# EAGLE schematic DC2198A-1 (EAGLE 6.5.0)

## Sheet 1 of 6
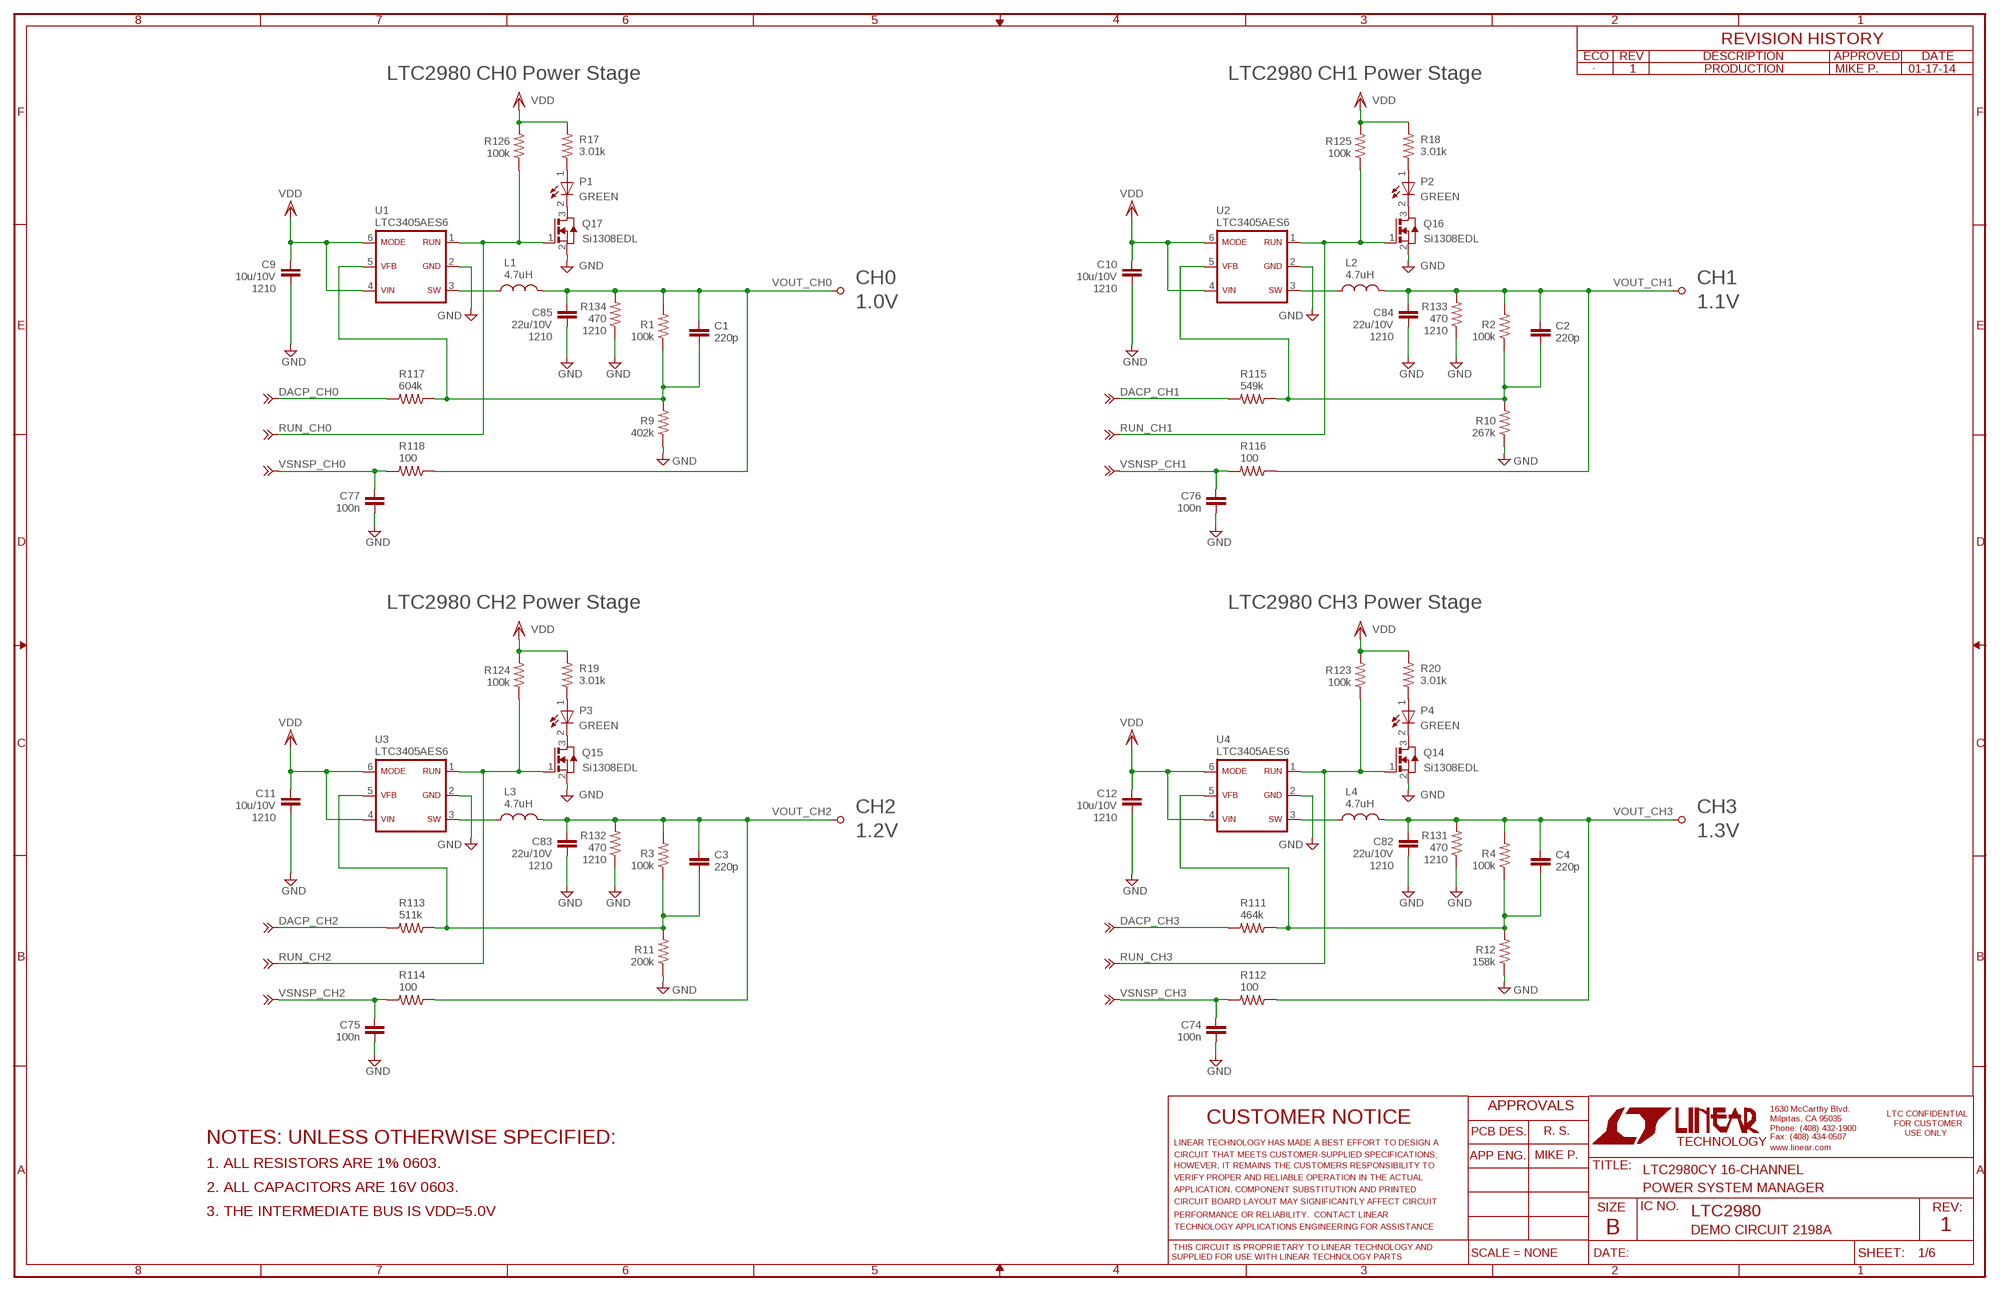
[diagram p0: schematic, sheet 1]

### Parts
C1  220p  CC0603_BOX  [C0603_BOX]
C2  220p  CC0603_BOX  [C0603_BOX]
C3  220p  CC0603_BOX  [C0603_BOX]
C4  220p  CC0603_BOX  [C0603_BOX]
C9  10u/10V  CC1210_BOX  [C1210_BOX]
C10  10u/10V  CC1210_BOX  [C1210_BOX]
C11  10u/10V  CC1210_BOX  [C1210_BOX]
C12  10u/10V  CC1210_BOX  [C1210_BOX]
C74  100n  CC0603_BOX  [C0603_BOX]
C75  100n  CC0603_BOX  [C0603_BOX]
C76  100n  CC0603_BOX  [C0603_BOX]
C77  100n  CC0603_BOX  [C0603_BOX]
C82  22u/10V  CC1210_BOX  [C1210_BOX]
C83  22u/10V  CC1210_BOX  [C1210_BOX]
C84  22u/10V  CC1210_BOX  [C1210_BOX]
C85  22u/10V  CC1210_BOX  [C1210_BOX]
L1  4.7uH  LL1210  [L1210]
L2  4.7uH  LL1210  [L1210]
L3  4.7uH  LL1210  [L1210]
L4  4.7uH  LL1210  [L1210]
P1  GREEN  LED-0603  [CHIPLED_0603]
P2  GREEN  LED-0603  [CHIPLED_0603]
P3  GREEN  LED-0603  [CHIPLED_0603]
P4  GREEN  LED-0603  [CHIPLED_0603]
Q14  Si1308EDL  SI1304  [SC70-3]
Q15  Si1308EDL  SI1304  [SC70-3]
Q16  Si1308EDL  SI1304  [SC70-3]
Q17  Si1308EDL  SI1304  [SC70-3]
R1  100k  RR0603_BOX  [R0603_BOX]
R2  100k  RR0603_BOX  [R0603_BOX]
R3  100k  RR0603_BOX  [R0603_BOX]
R4  100k  RR0603_BOX  [R0603_BOX]
R9  402k  RR0603_BOX  [R0603_BOX]
R10  267k  RR0603_BOX  [R0603_BOX]
R11  200k  RR0603_BOX  [R0603_BOX]
R12  158k  RR0603_BOX  [R0603_BOX]
R17  3.01k  RR0603_BOX  [R0603_BOX]
R18  3.01k  RR0603_BOX  [R0603_BOX]
R19  3.01k  RR0603_BOX  [R0603_BOX]
R20  3.01k  RR0603_BOX  [R0603_BOX]
R111  464k  RR0603_BOX  [R0603_BOX]
R112  100  RR0603_BOX  [R0603_BOX]
R113  511k  RR0603_BOX  [R0603_BOX]
R114  100  RR0603_BOX  [R0603_BOX]
R115  549k  RR0603_BOX  [R0603_BOX]
R116  100  RR0603_BOX  [R0603_BOX]
R117  604k  RR0603_BOX  [R0603_BOX]
R118  100  RR0603_BOX  [R0603_BOX]
R123  100k  RR0603_BOX  [R0603_BOX]
R124  100k  RR0603_BOX  [R0603_BOX]
R125  100k  RR0603_BOX  [R0603_BOX]
R126  100k  RR0603_BOX  [R0603_BOX]
R131  470  RR1210_BOX  [R1210_BOX]
R132  470  RR1210_BOX  [R1210_BOX]
R133  470  RR1210_BOX  [R1210_BOX]
R134  470  RR1210_BOX  [R1210_BOX]
TP3  TESTPOINT_BIG  [TP1]
TP4  TESTPOINT_BIG  [TP1]
TP5  TESTPOINT_BIG  [TP1]
TP6  TESTPOINT_BIG  [TP1]
U1  LTC3405AES6  LTC3405ES6  [SOT-23-6]
U2  LTC3405AES6  LTC3405ES6  [SOT-23-6]
U3  LTC3405AES6  LTC3405ES6  [SOT-23-6]
U4  LTC3405AES6  LTC3405ES6  [SOT-23-6]
VSNSN1  TESPOINT_SMD  TESPOINT_SMDVIA  [VIA]
VSNSN2  TESPOINT_SMD  TESPOINT_SMDVIA  [VIA]
VSNSN3  TESPOINT_SMD  TESPOINT_SMDVIA  [VIA]
VSNSN4  TESPOINT_SMD  TESPOINT_SMDVIA  [VIA]
VSNSN41  TESPOINT_SMD  TESPOINT_SMDVIA  [VIA]
VSNSN42  TESPOINT_SMD  TESPOINT_SMDVIA  [VIA]
VSNSN43  TESPOINT_SMD  TESPOINT_SMDVIA  [VIA]
VSNSN44  TESPOINT_SMD  TESPOINT_SMDVIA  [VIA]
VSNSN45  TESPOINT_SMD  TESPOINT_SMDVIA  [VIA]
VSNSN46  TESPOINT_SMD  TESPOINT_SMDVIA  [VIA]
VSNSN47  TESPOINT_SMD  TESPOINT_SMDVIA  [VIA]
VSNSN48  TESPOINT_SMD  TESPOINT_SMDVIA  [VIA]

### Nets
DACP_CH0: R117.2 VSNSN47.1 ; also sheet 5
DACP_CH1: R115.2 VSNSN45.1 ; also sheet 5
DACP_CH2: R113.2 VSNSN43.1 ; also sheet 5
DACP_CH3: R111.2 VSNSN41.1 ; also sheet 5
GND: C9.2 C10.2 C11.2 C12.2 C74.1 C75.1 C76.1 C77.1 C82.2 C83.2 C84.2 C85.2 Q14.2(S) Q15.2(S) Q16.2(S) Q17.2(S) R9.1 R10.1 R11.1 R12.1 R131.1 R132.1 R133.1 R134.1 U1.2 U2.2 U3.2 U4.2 ; also sheet 2,3,4,5,6
N$1: P1.P(A) R17.1
N$2: P1.N(C) Q17.3(D)
N$4: P2.P(A) R18.1
N$5: P2.N(C) Q16.3(D)
N$6: P3.P(A) R19.1
N$7: P3.N(C) Q15.3(D)
N$8: P4.P(A) R20.1
N$9: P4.N(C) Q14.3(D)
RUN_CH0: Q17.1(G) R126.1 U1.1 VSNSN1.1 ; also sheet 5
RUN_CH1: Q16.1(G) R125.1 U2.1 VSNSN2.1 ; also sheet 5
RUN_CH2: Q15.1(G) R124.1 U3.1 VSNSN3.1 ; also sheet 5
RUN_CH3: Q14.1(G) R123.1 U4.1 VSNSN4.1 ; also sheet 5
SW1: L1.1 U1.3
SW2: L2.1 U2.3
SW3: L3.1 U3.3
SW4: L4.1 U4.3
VDD: C9.1 C10.1 C11.1 C12.1 R17.2 R18.2 R19.2 R20.2 R123.2 R124.2 R125.2 R126.2 U1.4 U1.6 U2.4 U2.6 U3.4 U3.6 U4.4 U4.6 ; also sheet 2,3,4,5,6
VFB1: C1.2 R1.1 R9.2 R117.1 U1.5
VFB2: C2.2 R2.1 R10.2 R115.1 U2.5
VFB3: C3.2 R3.1 R11.2 R113.1 U3.5
VFB12: C4.2 R4.1 R12.2 R111.1 U4.5
VOUT_CH0: C1.1 C85.1 L1.2 R1.2 R118.1 R134.2 TP3.TP
VOUT_CH1: C2.1 C84.1 L2.2 R2.2 R116.1 R133.2 TP4.TP
VOUT_CH2: C3.1 C83.1 L3.2 R3.2 R114.1 R132.2 TP5.TP
VOUT_CH3: C4.1 C82.1 L4.2 R4.2 R112.1 R131.2 TP6.TP
VSNSP_CH0: C77.2 R118.2 VSNSN48.1 ; also sheet 5
VSNSP_CH1: C76.2 R116.2 VSNSN46.1 ; also sheet 5
VSNSP_CH2: C75.2 R114.2 VSNSN44.1 ; also sheet 5
VSNSP_CH3: C74.2 R112.2 VSNSN42.1 ; also sheet 5

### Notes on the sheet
- 1 | PRODUCTION | MIKE P. | 01-17-14
- LTC2980 CH0 Power Stage | LTC2980 CH1 Power Stage
- 1210 | CH0 | 1210 | CH1
- 1.0V | 1.1V
- 1210 | 1210
- 1210 | 1210
- LTC2980 CH2 Power Stage | LTC2980 CH3 Power Stage
- 1210 | CH2 | 1210 | CH3
- 1.2V | 1.3V
- 1210 | 1210
- 1210 | 1210
- R. S.
- NOTES: UNLESS OTHERWISE SPECIFIED:
- MIKE P.
- 1. ALL RESISTORS ARE 1% 0603.
- LTC2980CY 16-CHANNEL
- 2. ALL CAPACITORS ARE 16V 0603. | POWER SYSTEM MANAGER
- 3. THE INTERMEDIATE BUS IS VDD=5.0V | LTC2980
- DEMO CIRCUIT 2198A | 1

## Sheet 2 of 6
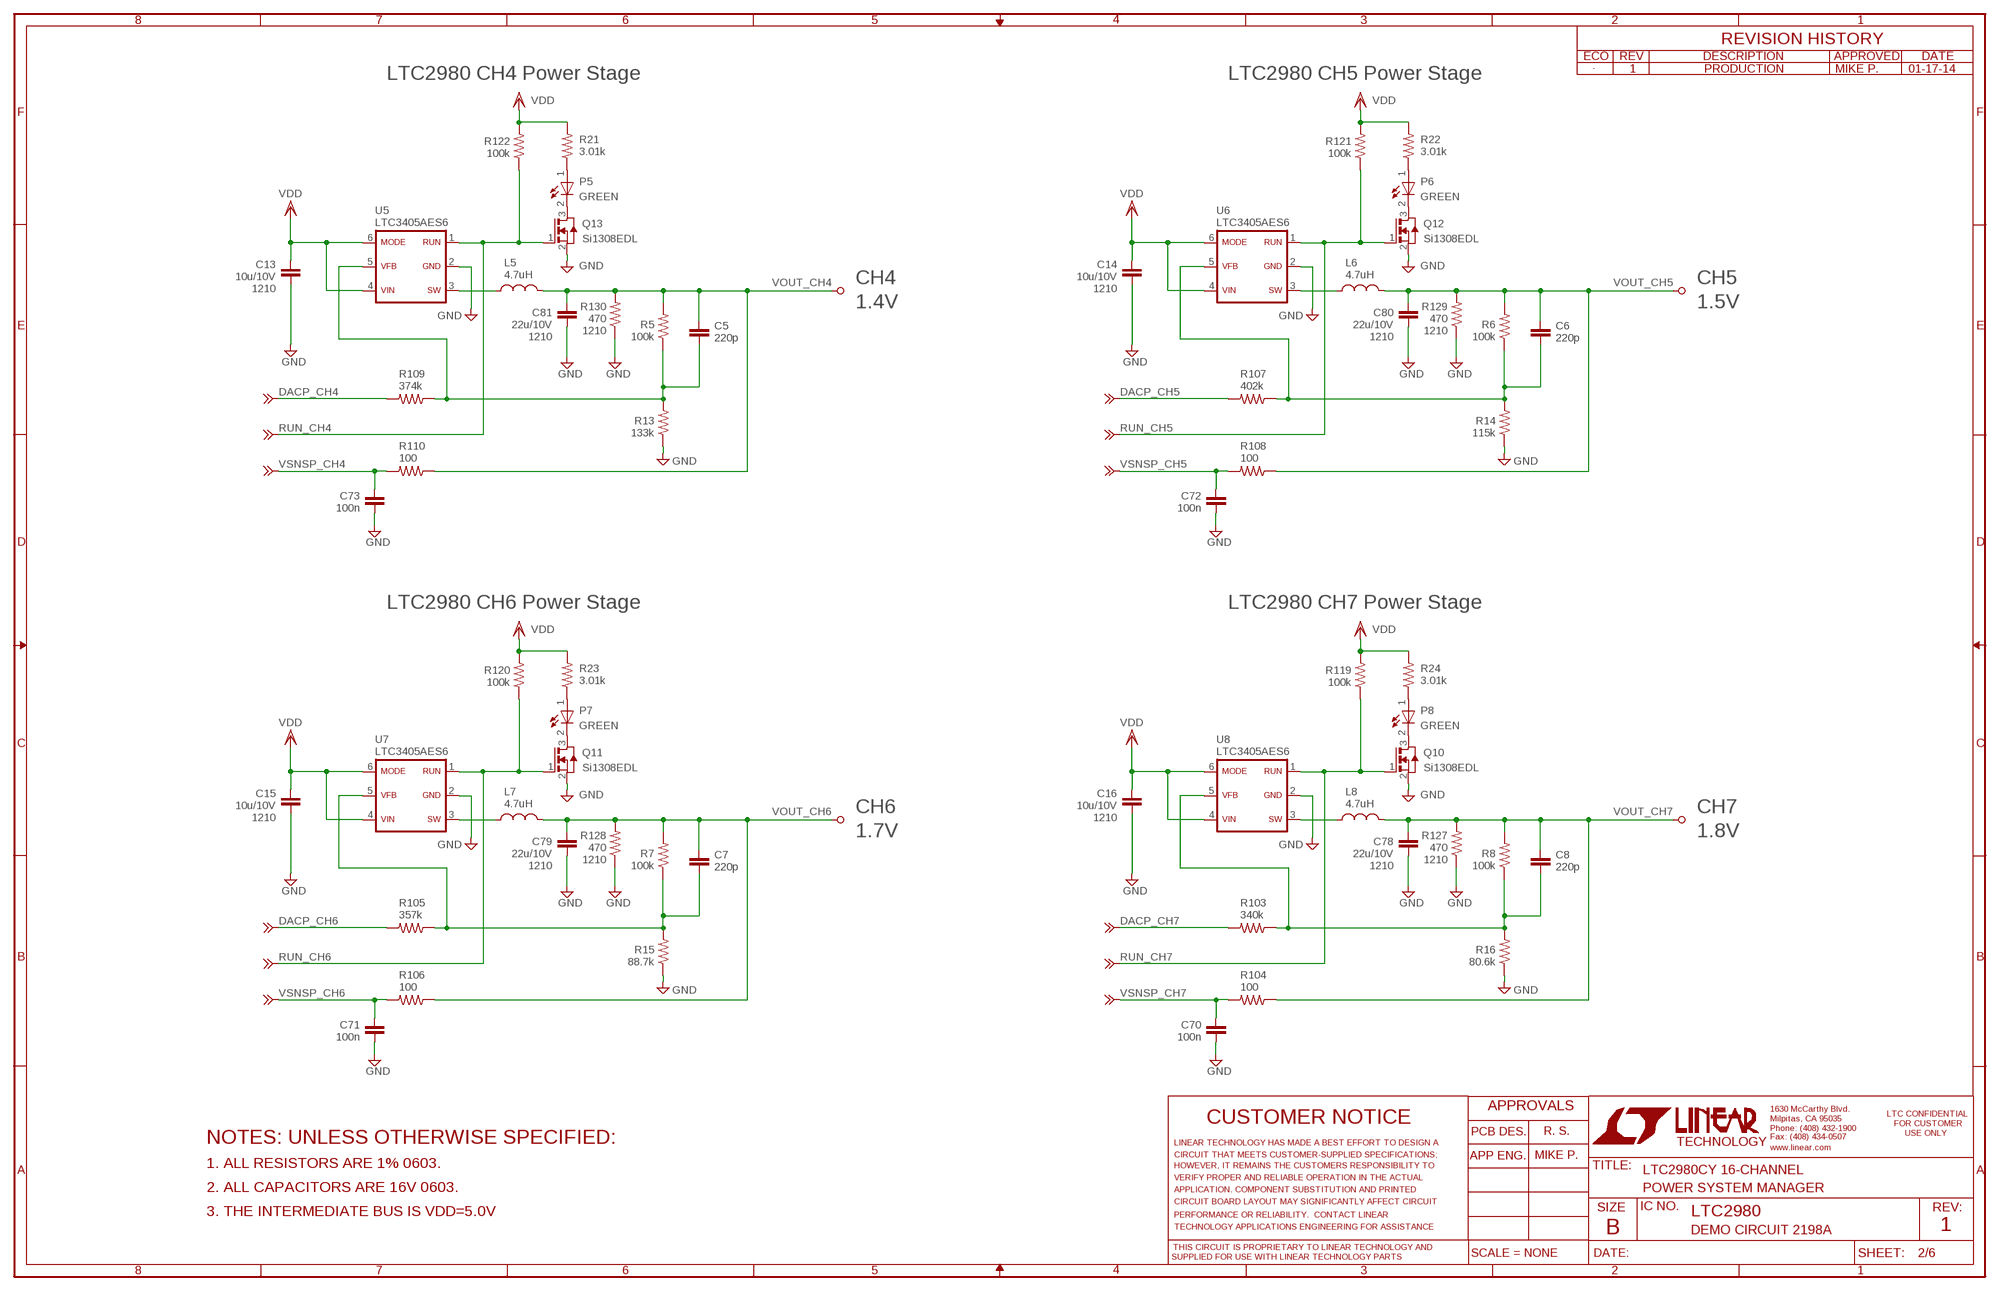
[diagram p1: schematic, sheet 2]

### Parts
C5  220p  CC0603_BOX  [C0603_BOX]
C6  220p  CC0603_BOX  [C0603_BOX]
C7  220p  CC0603_BOX  [C0603_BOX]
C8  220p  CC0603_BOX  [C0603_BOX]
C13  10u/10V  CC1210_BOX  [C1210_BOX]
C14  10u/10V  CC1210_BOX  [C1210_BOX]
C15  10u/10V  CC1210_BOX  [C1210_BOX]
C16  10u/10V  CC1210_BOX  [C1210_BOX]
C70  100n  CC0603_BOX  [C0603_BOX]
C71  100n  CC0603_BOX  [C0603_BOX]
C72  100n  CC0603_BOX  [C0603_BOX]
C73  100n  CC0603_BOX  [C0603_BOX]
C78  22u/10V  CC1210_BOX  [C1210_BOX]
C79  22u/10V  CC1210_BOX  [C1210_BOX]
C80  22u/10V  CC1210_BOX  [C1210_BOX]
C81  22u/10V  CC1210_BOX  [C1210_BOX]
L5  4.7uH  LL1210  [L1210]
L6  4.7uH  LL1210  [L1210]
L7  4.7uH  LL1210  [L1210]
L8  4.7uH  LL1210  [L1210]
P5  GREEN  LED-0603  [CHIPLED_0603]
P6  GREEN  LED-0603  [CHIPLED_0603]
P7  GREEN  LED-0603  [CHIPLED_0603]
P8  GREEN  LED-0603  [CHIPLED_0603]
Q10  Si1308EDL  SI1304  [SC70-3]
Q11  Si1308EDL  SI1304  [SC70-3]
Q12  Si1308EDL  SI1304  [SC70-3]
Q13  Si1308EDL  SI1304  [SC70-3]
R5  100k  RR0603_BOX  [R0603_BOX]
R6  100k  RR0603_BOX  [R0603_BOX]
R7  100k  RR0603_BOX  [R0603_BOX]
R8  100k  RR0603_BOX  [R0603_BOX]
R13  133k  RR0603_BOX  [R0603_BOX]
R14  115k  RR0603_BOX  [R0603_BOX]
R15  88.7k  RR0603_BOX  [R0603_BOX]
R16  80.6k  RR0603_BOX  [R0603_BOX]
R21  3.01k  RR0603_BOX  [R0603_BOX]
R22  3.01k  RR0603_BOX  [R0603_BOX]
R23  3.01k  RR0603_BOX  [R0603_BOX]
R24  3.01k  RR0603_BOX  [R0603_BOX]
R103  340k  RR0603_BOX  [R0603_BOX]
R104  100  RR0603_BOX  [R0603_BOX]
R105  357k  RR0603_BOX  [R0603_BOX]
R106  100  RR0603_BOX  [R0603_BOX]
R107  402k  RR0603_BOX  [R0603_BOX]
R108  100  RR0603_BOX  [R0603_BOX]
R109  374k  RR0603_BOX  [R0603_BOX]
R110  100  RR0603_BOX  [R0603_BOX]
R119  100k  RR0603_BOX  [R0603_BOX]
R120  100k  RR0603_BOX  [R0603_BOX]
R121  100k  RR0603_BOX  [R0603_BOX]
R122  100k  RR0603_BOX  [R0603_BOX]
R127  470  RR1210_BOX  [R1210_BOX]
R128  470  RR1210_BOX  [R1210_BOX]
R129  470  RR1210_BOX  [R1210_BOX]
R130  470  RR1210_BOX  [R1210_BOX]
TP7  TESTPOINT_BIG  [TP1]
TP8  TESTPOINT_BIG  [TP1]
TP9  TESTPOINT_BIG  [TP1]
TP10  TESTPOINT_BIG  [TP1]
U5  LTC3405AES6  LTC3405ES6  [SOT-23-6]
U6  LTC3405AES6  LTC3405ES6  [SOT-23-6]
U7  LTC3405AES6  LTC3405ES6  [SOT-23-6]
U8  LTC3405AES6  LTC3405ES6  [SOT-23-6]
VSNSN5  TESPOINT_SMD  TESPOINT_SMDVIA  [VIA]
VSNSN6  TESPOINT_SMD  TESPOINT_SMDVIA  [VIA]
VSNSN7  TESPOINT_SMD  TESPOINT_SMDVIA  [VIA]
VSNSN8  TESPOINT_SMD  TESPOINT_SMDVIA  [VIA]
VSNSN33  TESPOINT_SMD  TESPOINT_SMDVIA  [VIA]
VSNSN34  TESPOINT_SMD  TESPOINT_SMDVIA  [VIA]
VSNSN35  TESPOINT_SMD  TESPOINT_SMDVIA  [VIA]
VSNSN36  TESPOINT_SMD  TESPOINT_SMDVIA  [VIA]
VSNSN37  TESPOINT_SMD  TESPOINT_SMDVIA  [VIA]
VSNSN38  TESPOINT_SMD  TESPOINT_SMDVIA  [VIA]
VSNSN39  TESPOINT_SMD  TESPOINT_SMDVIA  [VIA]
VSNSN40  TESPOINT_SMD  TESPOINT_SMDVIA  [VIA]

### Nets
DACP_CH4: R109.2 VSNSN39.1 ; also sheet 5
DACP_CH5: R107.2 VSNSN37.1 ; also sheet 5
DACP_CH6: R105.2 VSNSN35.1 ; also sheet 5
DACP_CH7: R103.2 VSNSN33.1 ; also sheet 5
GND: C13.2 C14.2 C15.2 C16.2 C70.1 C71.1 C72.1 C73.1 C78.2 C79.2 C80.2 C81.2 Q10.2(S) Q11.2(S) Q12.2(S) Q13.2(S) R13.1 R14.1 R15.1 R16.1 R127.1 R128.1 R129.1 R130.1 U5.2 U6.2 U7.2 U8.2 ; also sheet 1,3,4,5,6
N$10: P5.P(A) R21.1
N$11: P5.N(C) Q13.3(D)
N$12: P6.P(A) R22.1
N$13: P6.N(C) Q12.3(D)
N$14: P7.P(A) R23.1
N$15: P7.N(C) Q11.3(D)
N$16: P8.P(A) R24.1
N$17: P8.N(C) Q10.3(D)
RUN_CH4: Q13.1(G) R122.1 U5.1 VSNSN5.1 ; also sheet 5
RUN_CH5: Q12.1(G) R121.1 U6.1 VSNSN6.1 ; also sheet 5
RUN_CH6: Q11.1(G) R120.1 U7.1 VSNSN7.1 ; also sheet 5
RUN_CH7: Q10.1(G) R119.1 U8.1 VSNSN8.1 ; also sheet 5
SW5: L5.1 U5.3
SW6: L6.1 U6.3
SW7: L7.1 U7.3
SW8: L8.1 U8.3
VDD: C13.1 C14.1 C15.1 C16.1 R21.2 R22.2 R23.2 R24.2 R119.2 R120.2 R121.2 R122.2 U5.4 U5.6 U6.4 U6.6 U7.4 U7.6 U8.4 U8.6 ; also sheet 1,3,4,5,6
VFB13: C5.2 R5.1 R13.2 R109.1 U5.5
VFB14: C6.2 R6.1 R14.2 R107.1 U6.5
VFB15: C7.2 R7.1 R15.2 R105.1 U7.5
VFB16: C8.2 R8.1 R16.2 R103.1 U8.5
VOUT_CH4: C5.1 C81.1 L5.2 R5.2 R110.1 R130.2 TP7.TP
VOUT_CH5: C6.1 C80.1 L6.2 R6.2 R108.1 R129.2 TP8.TP
VOUT_CH6: C7.1 C79.1 L7.2 R7.2 R106.1 R128.2 TP9.TP
VOUT_CH7: C8.1 C78.1 L8.2 R8.2 R104.1 R127.2 TP10.TP
VSNSP_CH4: C73.2 R110.2 VSNSN40.1 ; also sheet 5
VSNSP_CH5: C72.2 R108.2 VSNSN38.1 ; also sheet 5
VSNSP_CH6: C71.2 R106.2 VSNSN36.1 ; also sheet 5
VSNSP_CH7: C70.2 R104.2 VSNSN34.1 ; also sheet 5

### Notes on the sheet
- 1 | PRODUCTION | MIKE P. | 01-17-14
- LTC2980 CH4 Power Stage | LTC2980 CH5 Power Stage
- 1210 | CH4 | 1210 | CH5
- 1.4V | 1.5V
- 1210 | 1210
- 1210 | 1210
- LTC2980 CH6 Power Stage | LTC2980 CH7 Power Stage
- 1210 | CH6 | 1210 | CH7
- 1.7V | 1.8V
- 1210 | 1210
- 1210 | 1210
- R. S.
- NOTES: UNLESS OTHERWISE SPECIFIED:
- MIKE P.
- 1. ALL RESISTORS ARE 1% 0603.
- LTC2980CY 16-CHANNEL
- 2. ALL CAPACITORS ARE 16V 0603. | POWER SYSTEM MANAGER
- 3. THE INTERMEDIATE BUS IS VDD=5.0V | LTC2980
- DEMO CIRCUIT 2198A | 1

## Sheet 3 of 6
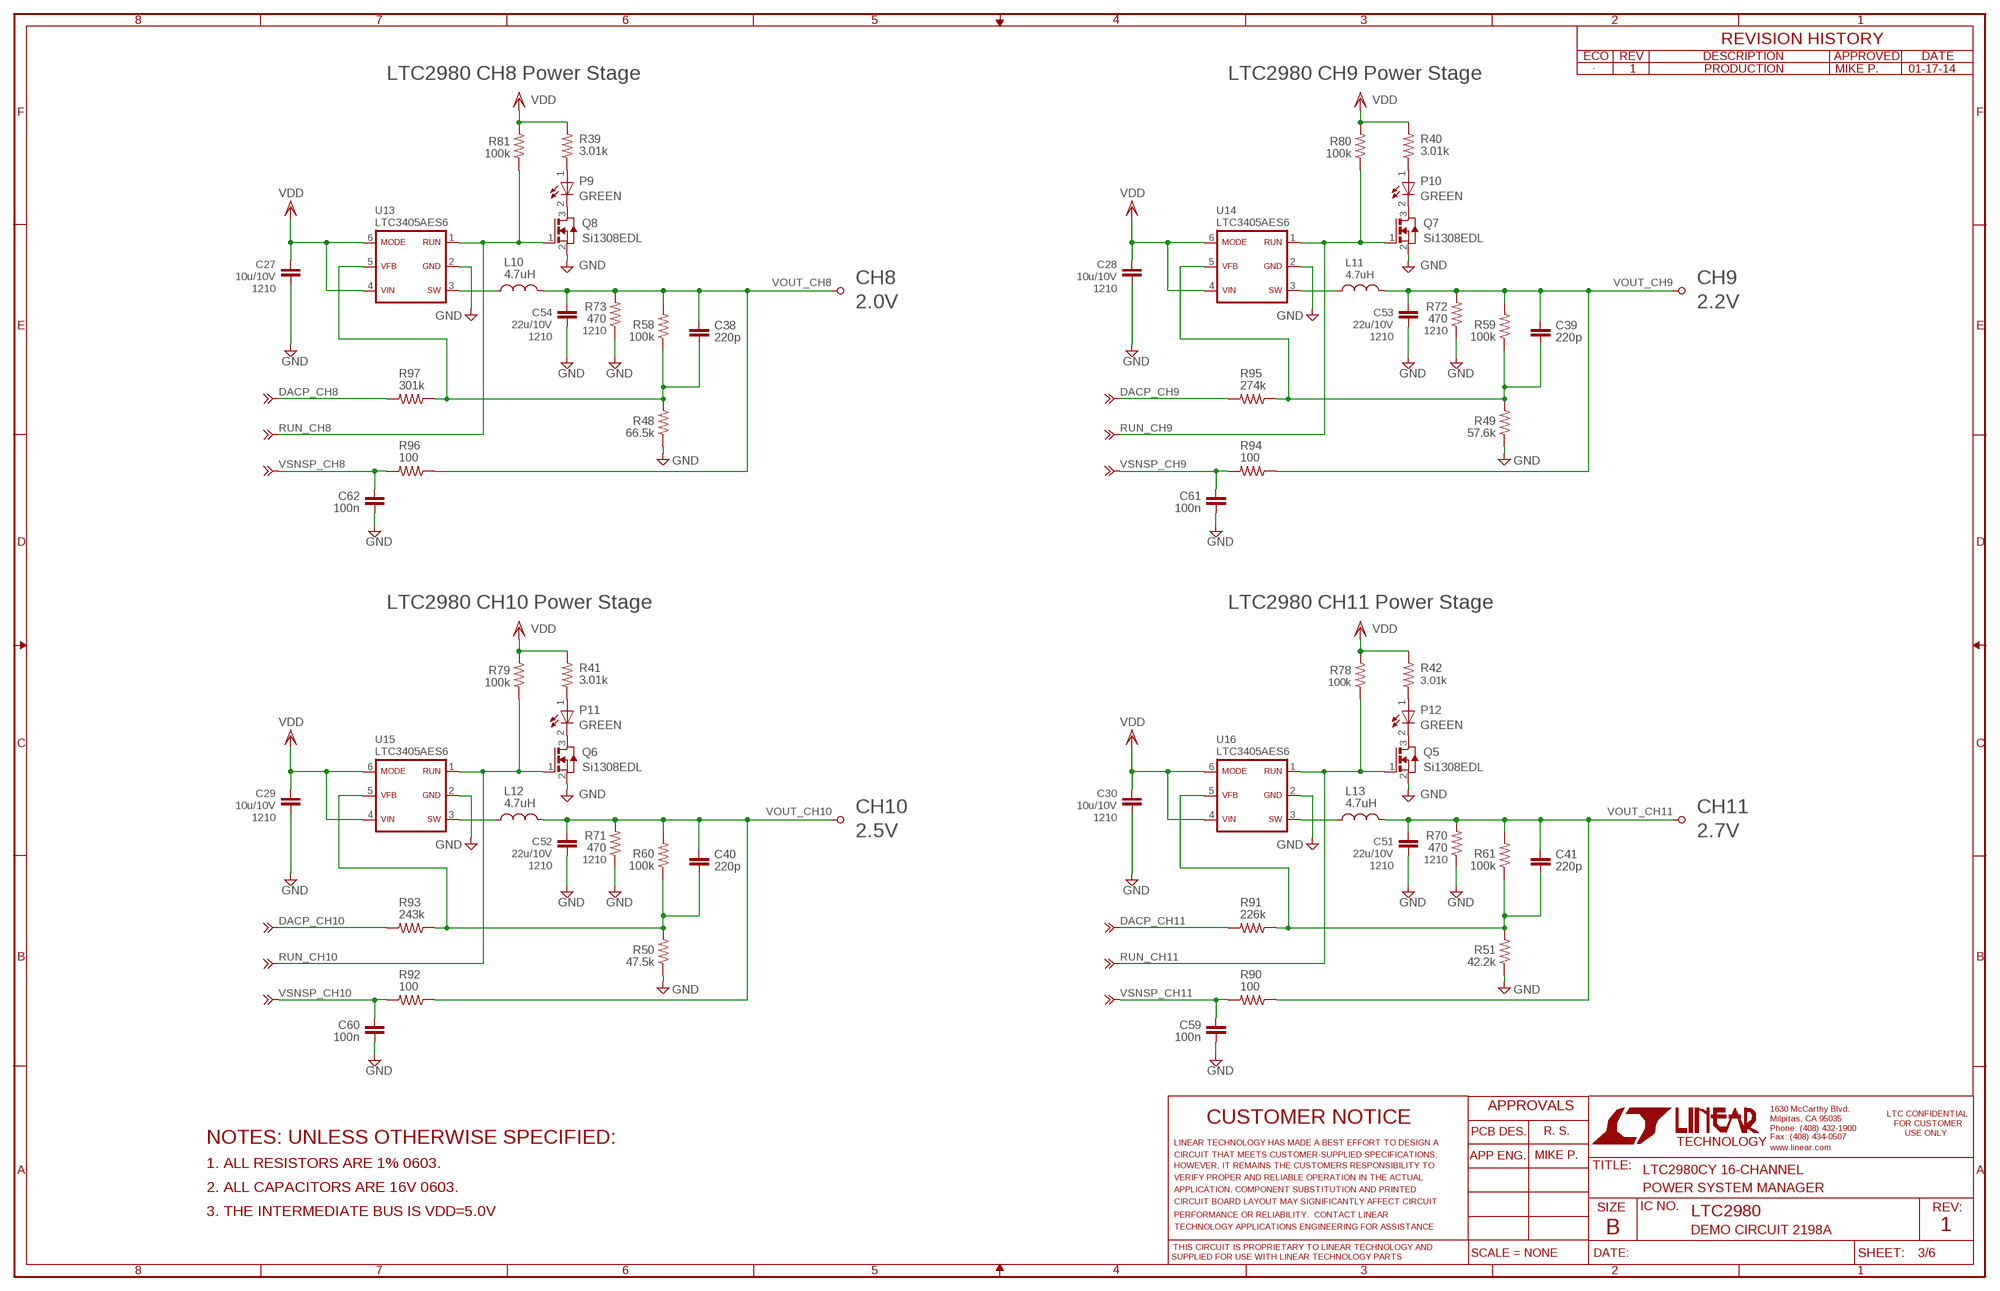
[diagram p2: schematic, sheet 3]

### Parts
C27  10u/10V  CC1210_BOX  [C1210_BOX]
C28  10u/10V  CC1210_BOX  [C1210_BOX]
C29  10u/10V  CC1210_BOX  [C1210_BOX]
C30  10u/10V  CC1210_BOX  [C1210_BOX]
C38  220p  CC0603_BOX  [C0603_BOX]
C39  220p  CC0603_BOX  [C0603_BOX]
C40  220p  CC0603_BOX  [C0603_BOX]
C41  220p  CC0603_BOX  [C0603_BOX]
C51  22u/10V  CC1210_BOX  [C1210_BOX]
C52  22u/10V  CC1210_BOX  [C1210_BOX]
C53  22u/10V  CC1210_BOX  [C1210_BOX]
C54  22u/10V  CC1210_BOX  [C1210_BOX]
C59  100n  CC0603_BOX  [C0603_BOX]
C60  100n  CC0603_BOX  [C0603_BOX]
C61  100n  CC0603_BOX  [C0603_BOX]
C62  100n  CC0603_BOX  [C0603_BOX]
L10  4.7uH  LL1210  [L1210]
L11  4.7uH  LL1210  [L1210]
L12  4.7uH  LL1210  [L1210]
L13  4.7uH  LL1210  [L1210]
P9  GREEN  LED-0603  [CHIPLED_0603]
P10  GREEN  LED-0603  [CHIPLED_0603]
P11  GREEN  LED-0603  [CHIPLED_0603]
P12  GREEN  LED-0603  [CHIPLED_0603]
Q5  Si1308EDL  SI1304  [SC70-3]
Q6  Si1308EDL  SI1304  [SC70-3]
Q7  Si1308EDL  SI1304  [SC70-3]
Q8  Si1308EDL  SI1304  [SC70-3]
R39  3.01k  RR0603_BOX  [R0603_BOX]
R40  3.01k  RR0603_BOX  [R0603_BOX]
R41  3.01k  RR0603_BOX  [R0603_BOX]
R42  3.01k  RR0603_BOX  [R0603_BOX]
R48  66.5k  RR0603_BOX  [R0603_BOX]
R49  57.6k  RR0603_BOX  [R0603_BOX]
R50  47.5k  RR0603_BOX  [R0603_BOX]
R51  42.2k  RR0603_BOX  [R0603_BOX]
R58  100k  RR0603_BOX  [R0603_BOX]
R59  100k  RR0603_BOX  [R0603_BOX]
R60  100k  RR0603_BOX  [R0603_BOX]
R61  100k  RR0603_BOX  [R0603_BOX]
R70  470  RR1210_BOX  [R1210_BOX]
R71  470  RR1210_BOX  [R1210_BOX]
R72  470  RR1210_BOX  [R1210_BOX]
R73  470  RR1210_BOX  [R1210_BOX]
R78  100k  RR0603_BOX  [R0603_BOX]
R79  100k  RR0603_BOX  [R0603_BOX]
R80  100k  RR0603_BOX  [R0603_BOX]
R81  100k  RR0603_BOX  [R0603_BOX]
R90  100  RR0603_BOX  [R0603_BOX]
R91  226k  RR0603_BOX  [R0603_BOX]
R92  100  RR0603_BOX  [R0603_BOX]
R93  243k  RR0603_BOX  [R0603_BOX]
R94  100  RR0603_BOX  [R0603_BOX]
R95  274k  RR0603_BOX  [R0603_BOX]
R96  100  RR0603_BOX  [R0603_BOX]
R97  301k  RR0603_BOX  [R0603_BOX]
TP23  TESTPOINT_BIG  [TP1]
TP24  TESTPOINT_BIG  [TP1]
TP25  TESTPOINT_BIG  [TP1]
TP26  TESTPOINT_BIG  [TP1]
U13  LTC3405AES6  LTC3405ES6  [SOT-23-6]
U14  LTC3405AES6  LTC3405ES6  [SOT-23-6]
U15  LTC3405AES6  LTC3405ES6  [SOT-23-6]
U16  LTC3405AES6  LTC3405ES6  [SOT-23-6]
VSNSN9  TESPOINT_SMD  TESPOINT_SMDVIA  [VIA]
VSNSN10  TESPOINT_SMD  TESPOINT_SMDVIA  [VIA]
VSNSN11  TESPOINT_SMD  TESPOINT_SMDVIA  [VIA]
VSNSN12  TESPOINT_SMD  TESPOINT_SMDVIA  [VIA]
VSNSN25  TESPOINT_SMD  TESPOINT_SMDVIA  [VIA]
VSNSN26  TESPOINT_SMD  TESPOINT_SMDVIA  [VIA]
VSNSN27  TESPOINT_SMD  TESPOINT_SMDVIA  [VIA]
VSNSN28  TESPOINT_SMD  TESPOINT_SMDVIA  [VIA]
VSNSN29  TESPOINT_SMD  TESPOINT_SMDVIA  [VIA]
VSNSN30  TESPOINT_SMD  TESPOINT_SMDVIA  [VIA]
VSNSN31  TESPOINT_SMD  TESPOINT_SMDVIA  [VIA]
VSNSN32  TESPOINT_SMD  TESPOINT_SMDVIA  [VIA]

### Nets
DACP_CH8: R97.2 VSNSN32.1 ; also sheet 5
DACP_CH9: R95.2 VSNSN30.1 ; also sheet 5
DACP_CH10: R93.2 VSNSN28.1 ; also sheet 5
DACP_CH11: R91.2 VSNSN26.1 ; also sheet 5
GND: C27.2 C28.2 C29.2 C30.2 C51.2 C52.2 C53.2 C54.2 C59.1 C60.1 C61.1 C62.1 Q5.2(S) Q6.2(S) Q7.2(S) Q8.2(S) R48.1 R49.1 R50.1 R51.1 R70.1 R71.1 R72.1 R73.1 U13.2 U14.2 U15.2 U16.2 ; also sheet 1,2,4,5,6
N$29: P9.P(A) R39.1
N$30: P9.N(C) Q8.3(D)
N$31: P10.P(A) R40.1
N$32: P10.N(C) Q7.3(D)
N$33: P11.P(A) R41.1
N$34: P11.N(C) Q6.3(D)
N$35: P12.P(A) R42.1
N$36: P12.N(C) Q5.3(D)
RUN_CH8: Q8.1(G) R81.1 U13.1 VSNSN9.1 ; also sheet 5
RUN_CH9: Q7.1(G) R80.1 U14.1 VSNSN10.1 ; also sheet 5
RUN_CH10: Q6.1(G) R79.1 U15.1 VSNSN11.1 ; also sheet 5
RUN_CH11: Q5.1(G) R78.1 U16.1 VSNSN12.1 ; also sheet 5
SW11: L10.1 U13.3
SW12: L11.1 U14.3
SW13: L12.1 U15.3
SW14: L13.1 U16.3
VDD: C27.1 C28.1 C29.1 C30.1 R39.2 R40.2 R41.2 R42.2 R78.2 R79.2 R80.2 R81.2 U13.4 U13.6 U14.4 U14.6 U15.4 U15.6 U16.4 U16.6 ; also sheet 1,2,4,5,6
VFB4: C38.2 R48.2 R58.1 R97.1 U13.5
VFB5: C39.2 R49.2 R59.1 R95.1 U14.5
VFB6: C40.2 R50.2 R60.1 R93.1 U15.5
VFB7: C41.2 R51.2 R61.1 R91.1 U16.5
VOUT_CH8: C38.1 C54.1 L10.2 R58.2 R73.2 R96.1 TP23.TP
VOUT_CH9: C39.1 C53.1 L11.2 R59.2 R72.2 R94.1 TP24.TP
VOUT_CH10: C40.1 C52.1 L12.2 R60.2 R71.2 R92.1 TP25.TP ; also sheet 5
VOUT_CH11: C41.1 C51.1 L13.2 R61.2 R70.2 R90.1 TP26.TP
VSNSP_CH8: C62.2 R96.2 VSNSN31.1 ; also sheet 5
VSNSP_CH9: C61.2 R94.2 VSNSN29.1 ; also sheet 5
VSNSP_CH10: C60.2 R92.2 VSNSN27.1 ; also sheet 5
VSNSP_CH11: C59.2 R90.2 VSNSN25.1 ; also sheet 5

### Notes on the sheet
- 1 | PRODUCTION | MIKE P. | 01-17-14
- LTC2980 CH8 Power Stage | LTC2980 CH9 Power Stage
- 1210 | CH8 | 1210 | CH9
- 2.0V | 2.2V
- 1210 | 1210
- 1210 | 1210
- LTC2980 CH10 Power Stage | LTC2980 CH11 Power Stage
- 1210 | CH10 | 1210 | CH11
- 2.5V | 2.7V
- 1210 | 1210
- 1210 | 1210
- R. S.
- NOTES: UNLESS OTHERWISE SPECIFIED:
- MIKE P.
- 1. ALL RESISTORS ARE 1% 0603.
- LTC2980CY 16-CHANNEL
- 2. ALL CAPACITORS ARE 16V 0603. | POWER SYSTEM MANAGER
- 3. THE INTERMEDIATE BUS IS VDD=5.0V | LTC2980
- DEMO CIRCUIT 2198A | 1

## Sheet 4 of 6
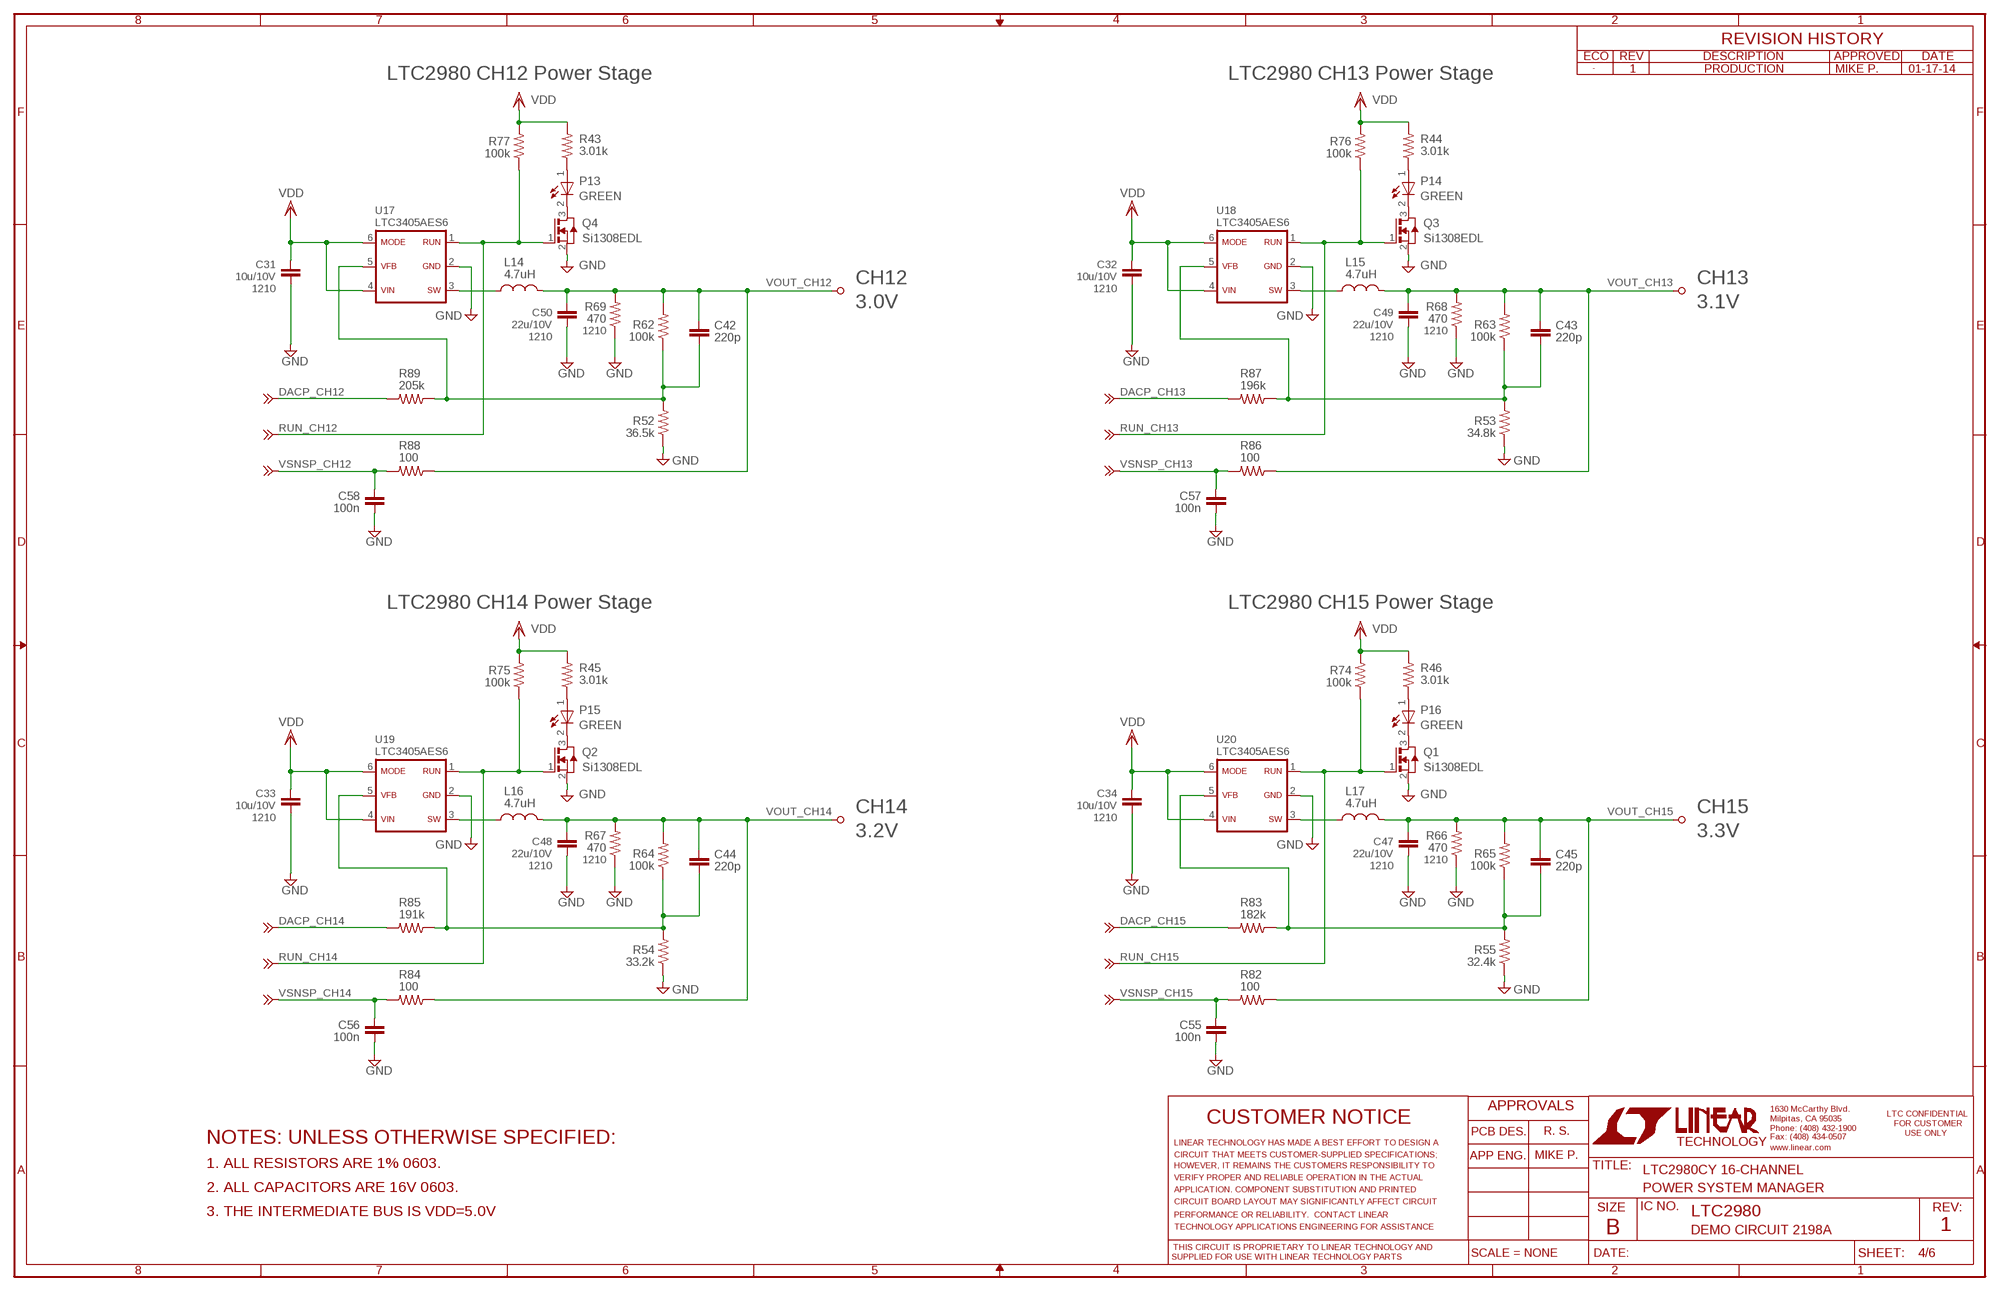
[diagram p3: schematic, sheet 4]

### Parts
C31  10u/10V  CC1210_BOX  [C1210_BOX]
C32  10u/10V  CC1210_BOX  [C1210_BOX]
C33  10u/10V  CC1210_BOX  [C1210_BOX]
C34  10u/10V  CC1210_BOX  [C1210_BOX]
C42  220p  CC0603_BOX  [C0603_BOX]
C43  220p  CC0603_BOX  [C0603_BOX]
C44  220p  CC0603_BOX  [C0603_BOX]
C45  220p  CC0603_BOX  [C0603_BOX]
C47  22u/10V  CC1210_BOX  [C1210_BOX]
C48  22u/10V  CC1210_BOX  [C1210_BOX]
C49  22u/10V  CC1210_BOX  [C1210_BOX]
C50  22u/10V  CC1210_BOX  [C1210_BOX]
C55  100n  CC0603_BOX  [C0603_BOX]
C56  100n  CC0603_BOX  [C0603_BOX]
C57  100n  CC0603_BOX  [C0603_BOX]
C58  100n  CC0603_BOX  [C0603_BOX]
L14  4.7uH  LL1210  [L1210]
L15  4.7uH  LL1210  [L1210]
L16  4.7uH  LL1210  [L1210]
L17  4.7uH  LL1210  [L1210]
P13  GREEN  LED-0603  [CHIPLED_0603]
P14  GREEN  LED-0603  [CHIPLED_0603]
P15  GREEN  LED-0603  [CHIPLED_0603]
P16  GREEN  LED-0603  [CHIPLED_0603]
Q1  Si1308EDL  SI1304  [SC70-3]
Q2  Si1308EDL  SI1304  [SC70-3]
Q3  Si1308EDL  SI1304  [SC70-3]
Q4  Si1308EDL  SI1304  [SC70-3]
R43  3.01k  RR0603_BOX  [R0603_BOX]
R44  3.01k  RR0603_BOX  [R0603_BOX]
R45  3.01k  RR0603_BOX  [R0603_BOX]
R46  3.01k  RR0603_BOX  [R0603_BOX]
R52  36.5k  RR0603_BOX  [R0603_BOX]
R53  34.8k  RR0603_BOX  [R0603_BOX]
R54  33.2k  RR0603_BOX  [R0603_BOX]
R55  32.4k  RR0603_BOX  [R0603_BOX]
R62  100k  RR0603_BOX  [R0603_BOX]
R63  100k  RR0603_BOX  [R0603_BOX]
R64  100k  RR0603_BOX  [R0603_BOX]
R65  100k  RR0603_BOX  [R0603_BOX]
R66  470  RR1210_BOX  [R1210_BOX]
R67  470  RR1210_BOX  [R1210_BOX]
R68  470  RR1210_BOX  [R1210_BOX]
R69  470  RR1210_BOX  [R1210_BOX]
R74  100k  RR0603_BOX  [R0603_BOX]
R75  100k  RR0603_BOX  [R0603_BOX]
R76  100k  RR0603_BOX  [R0603_BOX]
R77  100k  RR0603_BOX  [R0603_BOX]
R82  100  RR0603_BOX  [R0603_BOX]
R83  182k  RR0603_BOX  [R0603_BOX]
R84  100  RR0603_BOX  [R0603_BOX]
R85  191k  RR0603_BOX  [R0603_BOX]
R86  100  RR0603_BOX  [R0603_BOX]
R87  196k  RR0603_BOX  [R0603_BOX]
R88  100  RR0603_BOX  [R0603_BOX]
R89  205k  RR0603_BOX  [R0603_BOX]
TP27  TESTPOINT_BIG  [TP1]
TP28  TESTPOINT_BIG  [TP1]
TP29  TESTPOINT_BIG  [TP1]
TP30  TESTPOINT_BIG  [TP1]
U17  LTC3405AES6  LTC3405ES6  [SOT-23-6]
U18  LTC3405AES6  LTC3405ES6  [SOT-23-6]
U19  LTC3405AES6  LTC3405ES6  [SOT-23-6]
U20  LTC3405AES6  LTC3405ES6  [SOT-23-6]
VSNSN13  TESPOINT_SMD  TESPOINT_SMDVIA  [VIA]
VSNSN14  TESPOINT_SMD  TESPOINT_SMDVIA  [VIA]
VSNSN15  TESPOINT_SMD  TESPOINT_SMDVIA  [VIA]
VSNSN16  TESPOINT_SMD  TESPOINT_SMDVIA  [VIA]
VSNSN17  TESPOINT_SMD  TESPOINT_SMDVIA  [VIA]
VSNSN18  TESPOINT_SMD  TESPOINT_SMDVIA  [VIA]
VSNSN19  TESPOINT_SMD  TESPOINT_SMDVIA  [VIA]
VSNSN20  TESPOINT_SMD  TESPOINT_SMDVIA  [VIA]
VSNSN21  TESPOINT_SMD  TESPOINT_SMDVIA  [VIA]
VSNSN22  TESPOINT_SMD  TESPOINT_SMDVIA  [VIA]
VSNSN23  TESPOINT_SMD  TESPOINT_SMDVIA  [VIA]
VSNSN24  TESPOINT_SMD  TESPOINT_SMDVIA  [VIA]

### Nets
DACP_CH12: R89.2 VSNSN24.1 ; also sheet 5
DACP_CH13: R87.2 VSNSN22.1 ; also sheet 5
DACP_CH14: R85.2 VSNSN20.1 ; also sheet 5
DACP_CH15: R83.2 VSNSN18.1 ; also sheet 5
GND: C31.2 C32.2 C33.2 C34.2 C47.2 C48.2 C49.2 C50.2 C55.1 C56.1 C57.1 C58.1 Q1.2(S) Q2.2(S) Q3.2(S) Q4.2(S) R52.1 R53.1 R54.1 R55.1 R66.1 R67.1 R68.1 R69.1 U17.2 U18.2 U19.2 U20.2 ; also sheet 1,2,3,5,6
N$37: P13.P(A) R43.1
N$38: P13.N(C) Q4.3(D)
N$39: P14.P(A) R44.1
N$40: P14.N(C) Q3.3(D)
N$41: P15.P(A) R45.1
N$42: P15.N(C) Q2.3(D)
N$43: P16.P(A) R46.1
N$44: P16.N(C) Q1.3(D)
RUN_CH12: Q4.1(G) R77.1 U17.1 VSNSN13.1 ; also sheet 5
RUN_CH13: Q3.1(G) R76.1 U18.1 VSNSN14.1 ; also sheet 5
RUN_CH14: Q2.1(G) R75.1 U19.1 VSNSN15.1 ; also sheet 5
RUN_CH15: Q1.1(G) R74.1 U20.1 VSNSN16.1 ; also sheet 5
SW15: L14.1 U17.3
SW16: L15.1 U18.3
SW17: L16.1 U19.3
SW18: L17.1 U20.3
VDD: C31.1 C32.1 C33.1 C34.1 R43.2 R44.2 R45.2 R46.2 R74.2 R75.2 R76.2 R77.2 U17.4 U17.6 U18.4 U18.6 U19.4 U19.6 U20.4 U20.6 ; also sheet 1,2,3,5,6
VFB8: C42.2 R52.2 R62.1 R89.1 U17.5
VFB9: C43.2 R53.2 R63.1 R87.1 U18.5
VFB10: C44.2 R54.2 R64.1 R85.1 U19.5
VFB11: C45.2 R55.2 R65.1 R83.1 U20.5
VOUT_CH12: C42.1 C50.1 L14.2 R62.2 R69.2 R88.1 TP27.TP
VOUT_CH13: C43.1 C49.1 L15.2 R63.2 R68.2 R86.1 TP28.TP
VOUT_CH14: C44.1 C48.1 L16.2 R64.2 R67.2 R84.1 TP29.TP
VOUT_CH15: C45.1 C47.1 L17.2 R65.2 R66.2 R82.1 TP30.TP
VSNSP_CH12: C58.2 R88.2 VSNSN23.1 ; also sheet 5
VSNSP_CH13: C57.2 R86.2 VSNSN21.1 ; also sheet 5
VSNSP_CH14: C56.2 R84.2 VSNSN19.1 ; also sheet 5
VSNSP_CH15: C55.2 R82.2 VSNSN17.1 ; also sheet 5

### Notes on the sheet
- 1 | PRODUCTION | MIKE P. | 01-17-14
- LTC2980 CH12 Power Stage | LTC2980 CH13 Power Stage
- 1210 | CH12 | 1210 | CH13
- 3.0V | 3.1V
- 1210 | 1210
- 1210 | 1210
- LTC2980 CH14 Power Stage | LTC2980 CH15 Power Stage
- 1210 | CH14 | 1210 | CH15
- 3.2V | 3.3V
- 1210 | 1210
- 1210 | 1210
- R. S.
- NOTES: UNLESS OTHERWISE SPECIFIED:
- MIKE P.
- 1. ALL RESISTORS ARE 1% 0603.
- LTC2980CY 16-CHANNEL
- 2. ALL CAPACITORS ARE 16V 0603. | POWER SYSTEM MANAGER
- 3. THE INTERMEDIATE BUS IS VDD=5.0V | LTC2980
- DEMO CIRCUIT 2198A | 1

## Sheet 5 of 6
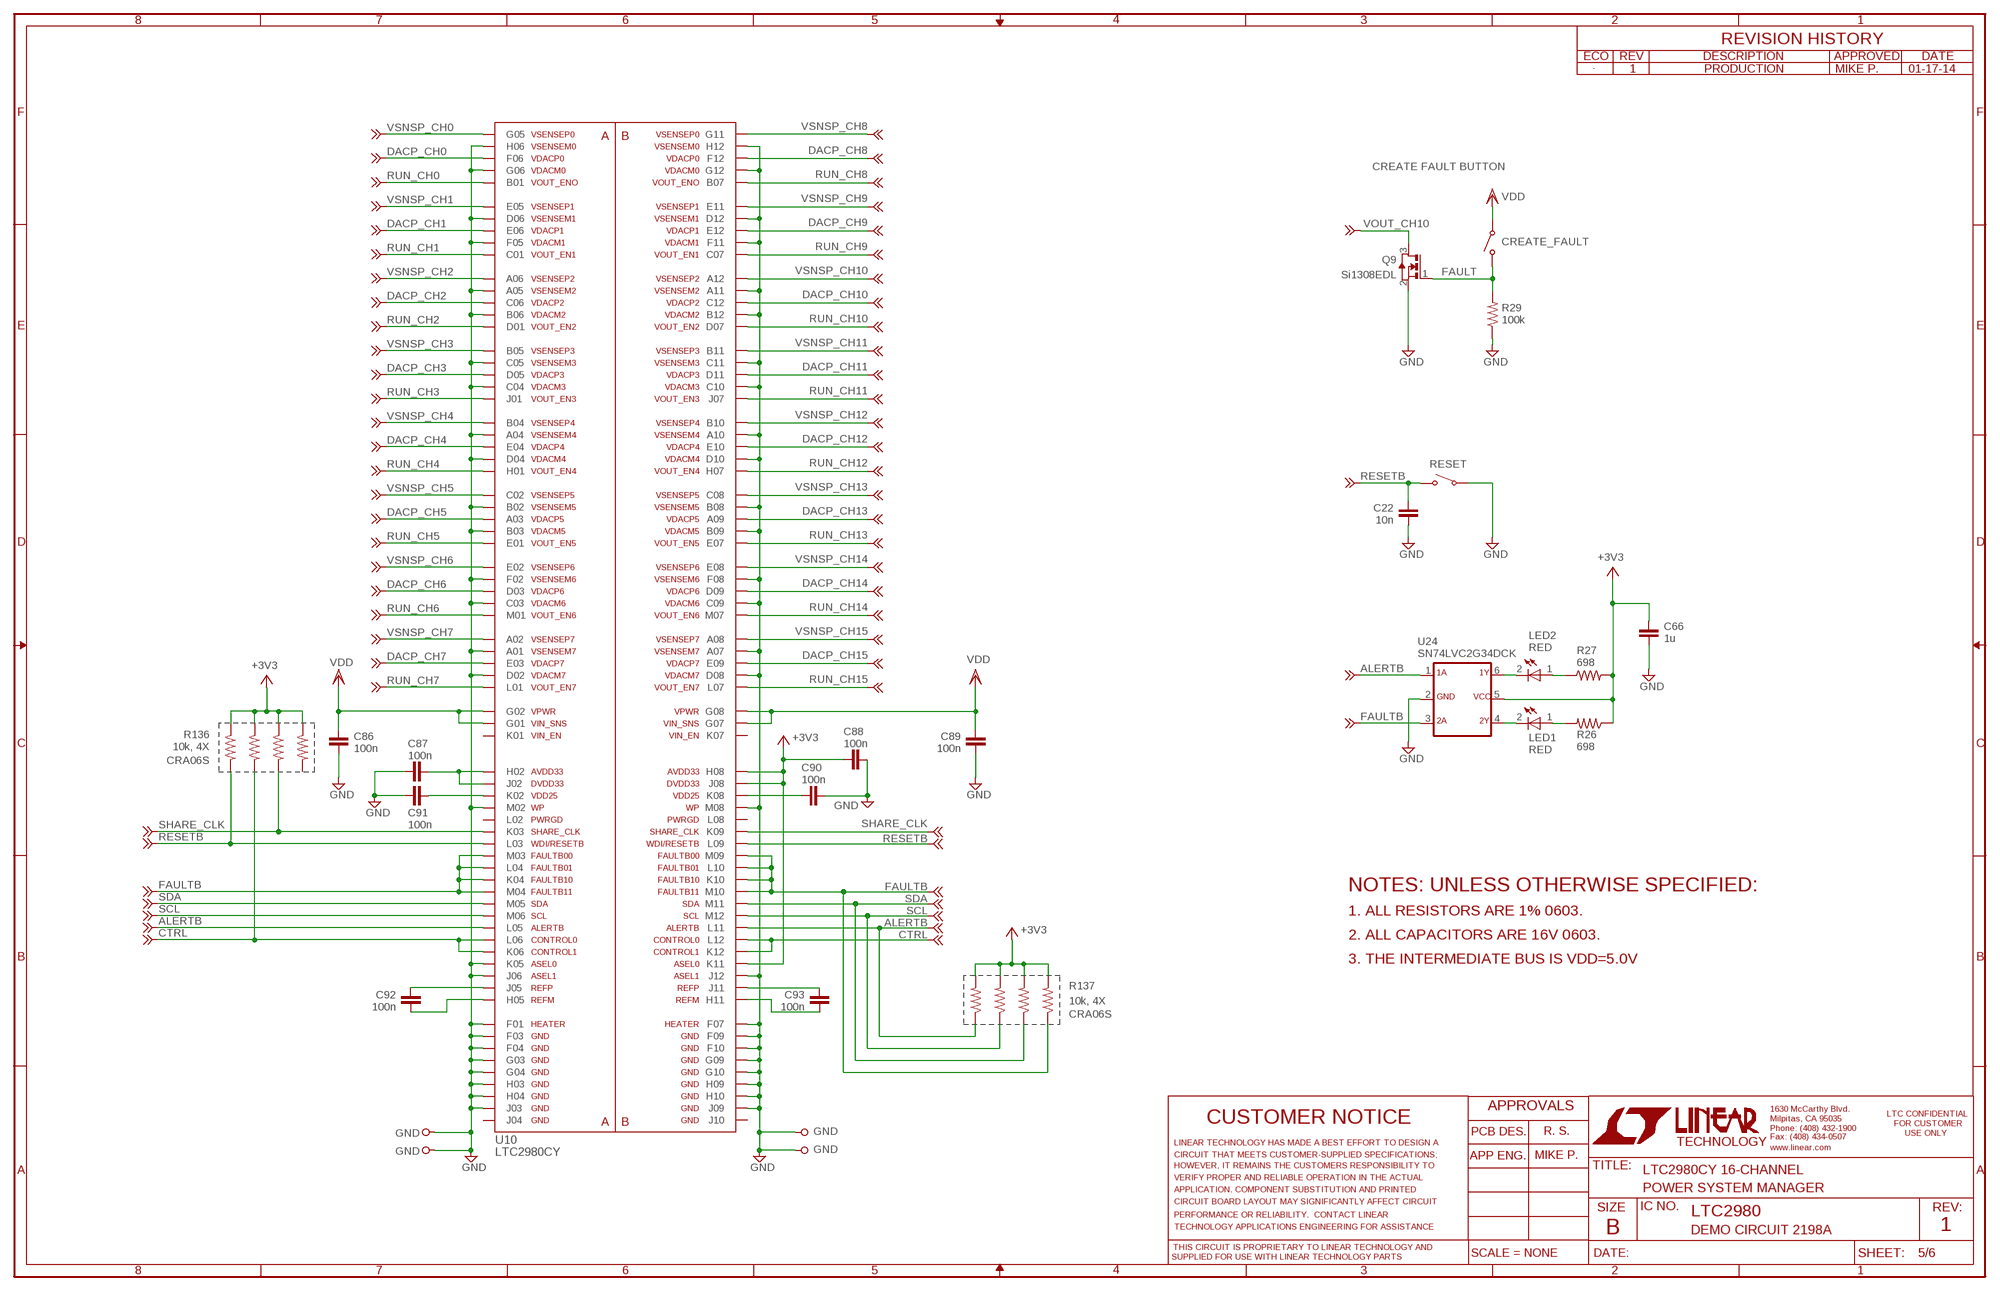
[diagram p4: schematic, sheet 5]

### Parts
C22  10n  CC0603_BOX  [C0603_BOX]
C66  1u  CC0603_BOX  [C0603_BOX]
C86  100n  CC0603_BOX  [C0603_BOX]
C87  100n  CC0603_BOX  [C0603_BOX]
C88  100n  CC0603_BOX  [C0603_BOX]
C89  100n  CC0603_BOX  [C0603_BOX]
C90  100n  CC0603_BOX  [C0603_BOX]
C91  100n  CC0603_BOX  [C0603_BOX]
C92  100n  CC0603_BOX  [C0603_BOX]
C93  100n  CC0603_BOX  [C0603_BOX]
LED1  RED  LED-0603  [CHIPLED_0603]
LED2  RED  LED-0603  [CHIPLED_0603]
Q9  Si1308EDL  SI1304  [SC70-3]
R26  698  RR0603_BOX  [R0603_BOX]
R27  698  RR0603_BOX  [R0603_BOX]
R29  100k  RR0603_BOX  [R0603_BOX]
R136  10k, 4X  R_ARRAY_4X_CRA06S  [R_VISHAY_CRA06S]
R137  10k, 4X  R_ARRAY_4X_CRA06S  [R_VISHAY_CRA06S]
SW1  PTS635SL25SMTR LFS  SWITCH_PTS635  [SWITCH_PTS635]
SW2  PTS635SK25SMTR LFS  SWITCH_PTS635  [SWITCH_PTS635]
TP15  TESTPOINT_BIG  [TP1]
TP16  TESTPOINT_BIG  [TP1]
TP17  TESTPOINT_BIG  [TP1]
TP18  TESTPOINT_BIG  [TP1]
U10  LTC2980CY  LTC2980  [BGA_144_1.0]
U24  SN74LVC2G34DCK  [SC70-6]

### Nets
+3V3: C66.1 C88.2 R26.1 R27.2 R136.R1_1 R136.R2_1 R136.R3_1 R136.R4_1 R137.R1_2 R137.R2_2 R137.R3_2 R137.R4_2 U10.H8(H08) U10.J8(J08) U10.K11 U24.5 ; also sheet 6
ALERTB: R137.R4_1 U10.L5(L05) U10.L11 U24.1 ; also sheet 6
CTRL: R136.R2_2 U10.K6(K06) U10.K12 U10.L6(L06) U10.L12 ; also sheet 6
DACP_CH0: U10.F6(F06) ; also sheet 1
DACP_CH1: U10.E6(E06) ; also sheet 1
DACP_CH2: U10.C6(C06) ; also sheet 1
DACP_CH3: U10.D5(D05) ; also sheet 1
DACP_CH4: U10.E4(E04) ; also sheet 2
DACP_CH5: U10.A3(A03) ; also sheet 2
DACP_CH6: U10.D3(D03) ; also sheet 2
DACP_CH7: U10.E3(E03) ; also sheet 2
DACP_CH8: U10.F12 ; also sheet 3
DACP_CH9: U10.E12 ; also sheet 3
DACP_CH10: U10.C12 ; also sheet 3
DACP_CH11: U10.D11 ; also sheet 3
DACP_CH12: U10.E10 ; also sheet 4
DACP_CH13: U10.A9(A09) ; also sheet 4
DACP_CH14: U10.D9(D09) ; also sheet 4
DACP_CH15: U10.E9(E09) ; also sheet 4
FAULT: Q9.1(G) R29.2 SW2.SW1 ; also sheet 6
FAULTB: R137.R1_1 U10.K4(K04) U10.K10 U10.L4(L04) U10.L10 U10.M3(M03) U10.M4(M04) U10.M9(M09) U10.M10 U24.3 ; also sheet 6
GND: C22.2 C66.2 C86.2 C87.2 C88.1 C89.2 C90.1 C91.1 Q9.2(S) R29.1 SW1.SW2 TP15.TP TP16.TP TP17.TP TP18.TP U10.A1(A01) U10.A4(A04) U10.A5(A05) U10.A7(A07) U10.A10 U10.A11 U10.B2(B02) U10.B3(B03) U10.B6(B06) U10.B8(B08) U10.B9(B09) U10.B12 U10.C3(C03) U10.C4(C04) U10.C5(C05) U10.C9(C09) U10.C10 U10.C11 U10.D2(D02) U10.D4(D04) U10.D6(D06) U10.D8(D08) U10.D10 U10.D12 U10.F1(F01) U10.F2(F02) U10.F3(F03) U10.F4(F04) U10.F5(F05) U10.F7(F07) U10.F8(F08) U10.F9(F09) U10.F10 U10.F11 U10.G3(G03) U10.G4(G04) U10.G6(G06) U10.G9(G09) U10.G10 U10.G12 U10.H3(H03) U10.H4(H04) U10.H6(H06) U10.H9(H09) U10.H10 U10.H12 U10.J3(J03) U10.J6(J06) U10.J9(J09) U10.J12 U10.K5(K05) U10.M2(M02) U10.M8(M08) U24.2 ; also sheet 1,2,3,4,6
N$3: LED1.P(A) R26.2
N$21: C90.2 U10.K8(K08)
N$22: C91.2 U10.K2(K02)
N$23: C92.1 U10.J5(J05)
N$24: C92.2 U10.H5(H05)
N$25: C93.1 U10.J11
N$26: C87.1 U10.H2(H02) U10.J2(J02)
N$27: C93.2 U10.H11
N$57: LED2.P(A) R27.1
N$58: LED1.N(C) U24.4
N$60: LED2.N(C) U24.6
RESETB: C22.1 R136.R1_2 SW1.SW1 U10.L3(L03) U10.L9(L09) ; also sheet 6
RUN_CH0: U10.B1(B01) ; also sheet 1
RUN_CH1: U10.C1(C01) ; also sheet 1
RUN_CH2: U10.D1(D01) ; also sheet 1
RUN_CH3: U10.J1(J01) ; also sheet 1
RUN_CH4: U10.H1(H01) ; also sheet 2
RUN_CH5: U10.E1(E01) ; also sheet 2
RUN_CH6: U10.M1(M01) ; also sheet 2
RUN_CH7: U10.L1(L01) ; also sheet 2
RUN_CH8: U10.B7(B07) ; also sheet 3
RUN_CH9: U10.C7(C07) ; also sheet 3
RUN_CH10: U10.D7(D07) ; also sheet 3
RUN_CH11: U10.J7(J07) ; also sheet 3
RUN_CH12: U10.H7(H07) ; also sheet 4
RUN_CH13: U10.E7(E07) ; also sheet 4
RUN_CH14: U10.M7(M07) ; also sheet 4
RUN_CH15: U10.L7(L07) ; also sheet 4
SCL: R137.R3_1 U10.M6(M06) U10.M12 ; also sheet 6
SDA: R137.R2_1 U10.M5(M05) U10.M11 ; also sheet 6
SHARE_CLK: R136.R3_2 U10.K3(K03) U10.K9(K09) ; also sheet 6
VDD: C86.1 C89.1 SW2.SW2 U10.G1(G01) U10.G2(G02) U10.G7(G07) U10.G8(G08) ; also sheet 1,2,3,4,6
VOUT_CH10: Q9.3(D) ; also sheet 3
VSNSP_CH0: U10.G5(G05) ; also sheet 1
VSNSP_CH1: U10.E5(E05) ; also sheet 1
VSNSP_CH2: U10.A6(A06) ; also sheet 1
VSNSP_CH3: U10.B5(B05) ; also sheet 1
VSNSP_CH4: U10.B4(B04) ; also sheet 2
VSNSP_CH5: U10.C2(C02) ; also sheet 2
VSNSP_CH6: U10.E2(E02) ; also sheet 2
VSNSP_CH7: U10.A2(A02) ; also sheet 2
VSNSP_CH8: U10.G11 ; also sheet 3
VSNSP_CH9: U10.E11 ; also sheet 3
VSNSP_CH10: U10.A12 ; also sheet 3
VSNSP_CH11: U10.B11 ; also sheet 3
VSNSP_CH12: U10.B10 ; also sheet 4
VSNSP_CH13: U10.C8(C08) ; also sheet 4
VSNSP_CH14: U10.E8(E08) ; also sheet 4
VSNSP_CH15: U10.A8(A08) ; also sheet 4
Unconnected: R136.R4_2 U10.J4(J04) U10.J10 U10.K1(K01) U10.K7(K07) U10.L2(L02) U10.L8(L08)

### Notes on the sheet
- 1 | PRODUCTION | MIKE P. | 01-17-14
- CREATE FAULT BUTTON
- CREATE_FAULT
- RESET
- CRA06S
- NOTES: UNLESS OTHERWISE SPECIFIED:
- 1. ALL RESISTORS ARE 1% 0603.
- 2. ALL CAPACITORS ARE 16V 0603.
- 3. THE INTERMEDIATE BUS IS VDD=5.0V
- CRA06S
- R. S.
- MIKE P.
- LTC2980CY 16-CHANNEL
- POWER SYSTEM MANAGER
- LTC2980
- DEMO CIRCUIT 2198A | 1

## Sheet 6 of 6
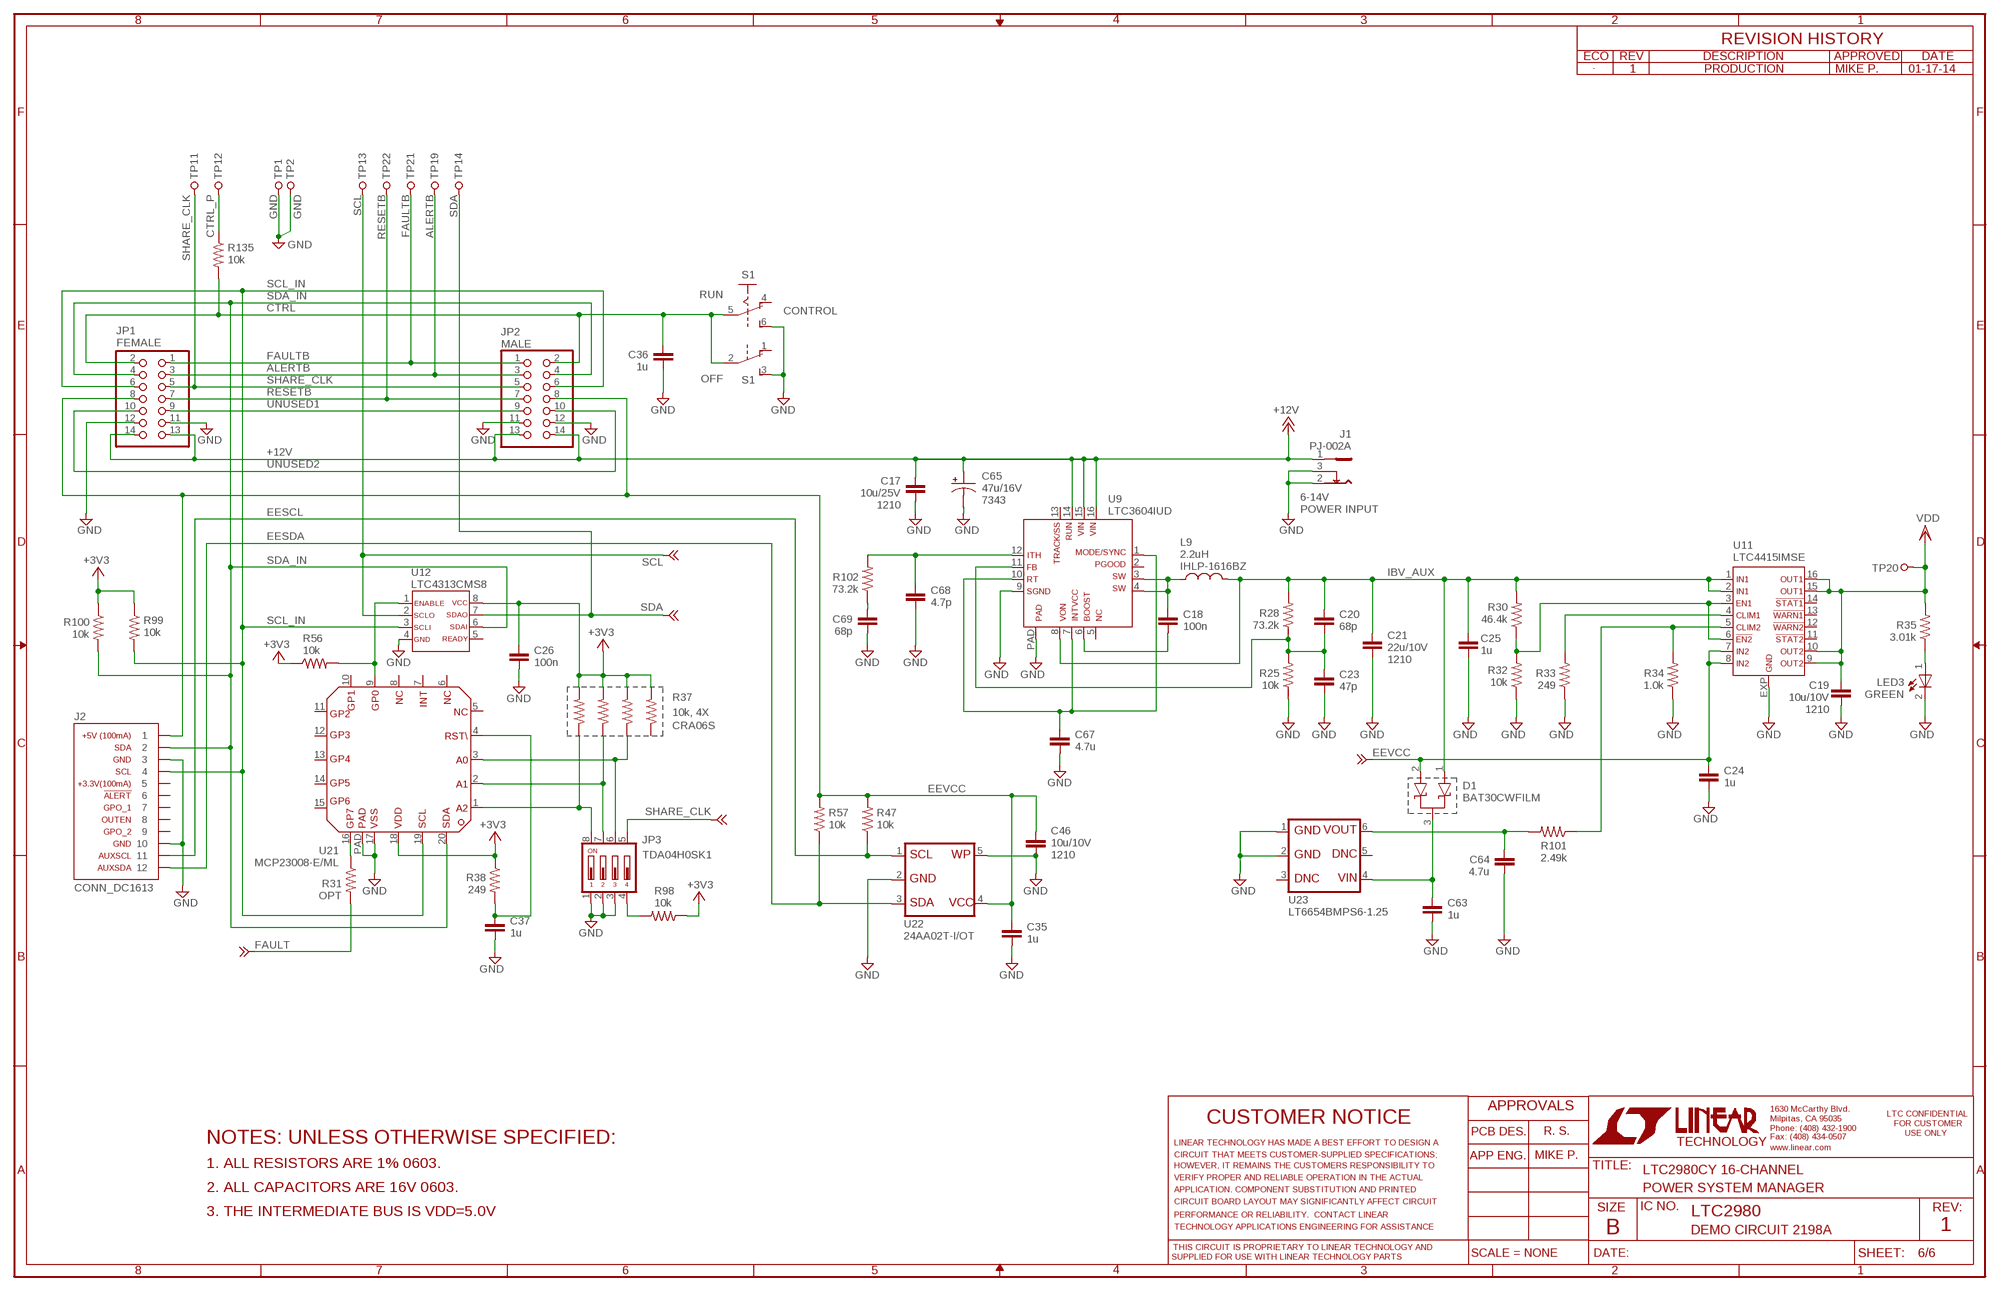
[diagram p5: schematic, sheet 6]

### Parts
C17  10u/25V  CC1210_BOX  [C1210_BOX]
C18  100n  CC0603_BOX  [C0603_BOX]
C19  10u/10V  CC1210_BOX  [C1210_BOX]
C20  68p  CC0603_BOX  [C0603_BOX]
C21  22u/10V  CC1210_BOX  [C1210_BOX]
C23  47p  CC0603_BOX  [C0603_BOX]
C24  1u  CC0603_BOX  [C0603_BOX]
C25  1u  CC0603_BOX  [C0603_BOX]
C26  100n  CC0603_BOX  [C0603_BOX]
C35  1u  CC0603_BOX  [C0603_BOX]
C36  1u  CC0603_BOX  [C0603_BOX]
C37  1u  CC0603_BOX  [C0603_BOX]
C46  10u/10V  CC1210_BOX  [C1210_BOX]
C63  1u  CC0603_BOX  [C0603_BOX]
C64  4.7u  CC0603_BOX  [C0603_BOX]
C65  47u/16V  CPOL  [C7343]
C67  4.7u  CC0603_BOX  [C0603_BOX]
C68  4.7p  CC0603_BOX  [C0603_BOX]
C69  68p  CC0603_BOX  [C0603_BOX]
D1  BAT30CWFILM  [SC70-3]
J1  PJ-002A  [PJ-002A]
J2  CONN_DC1613  [CONN_DC1613]
JP1  FEMALE  PINHD-2X07_2.00  [2X07M]
JP2  MALE  PINHD-2X07_2.00  [2X07M]
JP3  TDA04H0SK1  [SMT_DIP_4]
L9  2.2uH  LVISHAY-IHLP1616AB  [IHLP_1616AB]
LED3  GREEN  LED-0603  [CHIPLED_0603]
R25  10k  RR0603_BOX  [R0603_BOX]
R28  73.2k  RR0603_BOX  [R0603_BOX]
R30  46.4k  RR0603_BOX  [R0603_BOX]
R31  OPT  RR0603_BOX  [R0603_BOX]
R32  10k  RR0603_BOX  [R0603_BOX]
R33  249  RR0603_BOX  [R0603_BOX]
R34  1.0k  RR0603_BOX  [R0603_BOX]
R35  3.01k  RR0603_BOX  [R0603_BOX]
R37  10k, 4X  R_ARRAY_4X_CRA06S  [R_VISHAY_CRA06S]
R38  249  RR0603_BOX  [R0603_BOX]
R47  10k  RR0603_BOX  [R0603_BOX]
R56  10k  RR0603_BOX  [R0603_BOX]
R57  10k  RR0603_BOX  [R0603_BOX]
R98  10k  RR0603_BOX  [R0603_BOX]
R99  10k  RR0603_BOX  [R0603_BOX]
R100  10k  RR0603_BOX  [R0603_BOX]
R101  2.49k  RR0603_BOX  [R0603_BOX]
R102  73.2k  RR0603_BOX  [R0603_BOX]
R135  10k  RR0603_BOX  [R0603_BOX]
S1  CONTROL  JS202011CQN  [JS202011CQN]
TP1  TESTPOINT_BIG  [TP1]
TP2  TESTPOINT_BIG  [TP1]
TP11  TESTPOINT_BIG  [TP1]
TP12  TESTPOINT_BIG  [TP1]
TP13  TESTPOINT_BIG  [TP1]
TP14  TESTPOINT_BIG  [TP1]
TP19  TESTPOINT_BIG  [TP1]
TP20  TURRET_SMALL_2308TP  [TURRET_SMALL_2308]
TP21  TESTPOINT_BIG  [TP1]
TP22  TESTPOINT_BIG  [TP1]
U9  LTC3604IUD  [QFN16_3X3]
U11  LTC4415IMSE  [MSOP16_EXP]
U12  LTC4313CMS8  [MSOP-8]
U21  MCP23008-E/ML  [QFN20]
U22  24AA02T-I/OT  24AA64  [SOT-23-5]
U23  LT6654BMPS6-1.25  LTC6654SOT23-6  [SOT-23-6@1]

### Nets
+3V3: C26.1 R37.R1_2 R37.R2_2 R37.R3_2 R37.R4_2 R38.1 R56.1 R98.1 R99.1 R100.1 U12.8 U21.18 ; also sheet 5
+12V: C17.2 C65.+ J1.1 JP1.13 JP1.14 JP2.13 JP2.14 U9.14 U9.15 U9.16
A0_MUX: JP3.6 R37.R2_1 U21.3
A1_MUX: JP3.7 R37.R3_1 U21.2
A2_MUX: JP3.8 R37.R4_1 U21.1
ALERTB: JP1.3 JP2.3 TP19.TP ; also sheet 5
CTRL: C36.1 JP1.2 JP2.2 R135.2 S1.2(B:P) S1.5(A:P) ; also sheet 5
CTRL_P: R135.1 TP12.TP
EESCL: J2.11 R47.1 U22.1
EESDA: J2.12 R57.1 U22.3
EEVCC: C24.1 C35.1 C46.1 D1.2 J2.1 JP1.8 JP2.8 R47.2 R57.2 U11.7 U11.8 U22.4
FAULT: R31.2 ; also sheet 5
FAULTB: JP1.1 JP2.1 TP21.TP ; also sheet 5
FB_LTC3604: C20.2 C23.1 R25.2 R28.1 U9.11
GND: C17.1 C19.2 C21.2 C23.2 C24.2 C25.2 C26.2 C35.2 C36.2 C37.2 C46.2 C63.2 C64.1 C65.- C67.2 C68.2 C69.2 J1.2 J1.3 J2.3 J2.10 JP1.11 JP1.12 JP2.11 JP2.12 JP3.1 JP3.2 JP3.3 LED3.N(C) R25.1 R32.1 R33.1 R34.1 S1.3(B:S) S1.6(A:S) TP1.TP TP2.TP U9.9 U9.PAD U11.EXP U12.4 U21.17 U21.PAD U22.2 U22.5 U23.1 U23.2 ; also sheet 1,2,3,4,5
IBV_AUX: C20.1 C21.1 C25.1 D1.1 L9.2 R28.2 R30.2 U9.8 U11.1 U11.2
INTVCC_LTC3604: C67.1 U9.1 U9.7 U9.10
ITH_LTC3604: C68.1 R102.2 U9.12
N$18: R31.1 U21.16
N$19: C63.1 D1.3 U23.4
N$20: JP3.4 R98.2
N$61: C69.1 R102.1
N$63: LED3.P(A) R35.1
N$64: R34.2 R101.1 U11.5
N$66: C37.1 R38.2 U21.4
N$68: R33.2 U11.4
N$69: R30.1 R32.2 U11.3 U11.6
N$70: C18.2 U9.6
N$74: R56.2 U12.1 U21.9
RESETB: JP1.7 JP2.7 TP22.TP ; also sheet 5
SCL: TP13.TP U12.2 ; also sheet 5
SCL_IN: J2.4 JP1.6 JP2.6 R99.2 U12.3 U21.19
SDA: TP14.TP U12.7 ; also sheet 5
SDA_IN: J2.2 JP1.4 JP2.4 R100.2 U12.6 U21.20
SHARE_CLK: JP1.5 JP2.5 JP3.5 TP11.TP ; also sheet 5
SW_LTC3604: C18.1 L9.1 U9.3 U9.4
UNUSED1: JP1.9 JP2.9
UNUSED2: JP1.10 JP2.10
VDD: C19.1 R35.2 TP20.TP1 U11.9 U11.10 U11.15 U11.16 ; also sheet 1,2,3,4,5
VREF: C64.2 R101.2 U23.6
Unconnected: J2.5 J2.6 J2.7 J2.8 J2.9 R37.R1_1 S1.1(B:O) S1.4(A:O) U9.2 U9.5 U9.13 U11.11 U11.12 U11.13 U11.14 U12.5 U21.5 U21.6 U21.7 U21.8 U21.10 U21.11 U21.12 U21.13 U21.14 U21.15 U23.3 U23.5

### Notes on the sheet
- 1 | PRODUCTION | MIKE P. | 01-17-14
- RUN
- OFF
- 1210 | 7343 | 6-14V
- POWER INPUT
- IHLP-1616BZ
- 1210
- 1210
- CRA06S
- 1210
- R. S.
- NOTES: UNLESS OTHERWISE SPECIFIED:
- MIKE P.
- 1. ALL RESISTORS ARE 1% 0603.
- LTC2980CY 16-CHANNEL
- 2. ALL CAPACITORS ARE 16V 0603. | POWER SYSTEM MANAGER
- 3. THE INTERMEDIATE BUS IS VDD=5.0V | LTC2980
- DEMO CIRCUIT 2198A | 1

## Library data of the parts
C1-C64 C66-C93 = kalin:C: CAPACITOR, European symbol
C65 = kalin:CPOL: Polarized Capacitor
D1 = kalin:BAT30CWFILM: Small signal dual schottky diode (common cathode)
J1 = kalin:PJ-002A
J2 = kalin:CONN_DC1613: Connector for LT DC1613 USB Dongle
JP1 JP2 = pinhead_2mm:PINHD-2X07: PIN HEADER
JP3 = kalin:TDA04H0SK1: Ultra-miniature Surface Mount Half-pitch DIP Switch
L1-L17 = kalin:L: Inductor
LED1-LED3 P1-P16 = kalin:LED-0603: SMD LED in R0603
Q1-Q17 = kalin:SI1304: N-Channel 30 V (D-S) MOSFET
R1-R35 R38-R135 = kalin:R: RESISTOR, American symbol
R37 R136 R137 = kalin:R_ARRAY_4X_CRA06S: Thick Film Resistor Array
S1 = kalin:JS202011CQN: SLIDING SWITCH Siemens, distributor Buerklin, 11G766
SW1 SW2 = kalin:SWITCH_PTS635: PTS635SL25 Surface Mount Tactile Switch
TP1-TP19 TP21-TP30 = kalin:TESTPOINT_BIG: Large Test Point
TP20 = kalin:TURRET_SMALL_2308: Small Test Turret Mill-Max 2308
U1-U8 U13-U20 = kalin:LTC3405: 1.5MHz, 300mA Synchronous Step-Down Regulator in ThinSOT
U9 = kalin:LTC3604: 2.5A, 15V Monolithic Synchronous Step-Down Regulator
U10 = kalin:LTC2980
U11 = kalin:LTC4415: Dual 4A Ideal Diodes with Adjustable Current Limit
U12 = kalin:LTC4313: 2-Wire Bus Buffers with High Noise Margin
U21 = kalin:MCP23008: I2C 8-pin IO Expander
U22 = kalin:24AA64: 64Kbit I2C Serial EEPROM
U23 = kalin:LTC6654: SOT-23 Precision Wide Supply High Output Drive Low Noise Reference
U24 = kalin:SN74LVC2G34: Dual Buffer Gate
VSNSN1-VSNSN48 = kalin:TESPOINT_SMD: SMALL SMD Test Point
